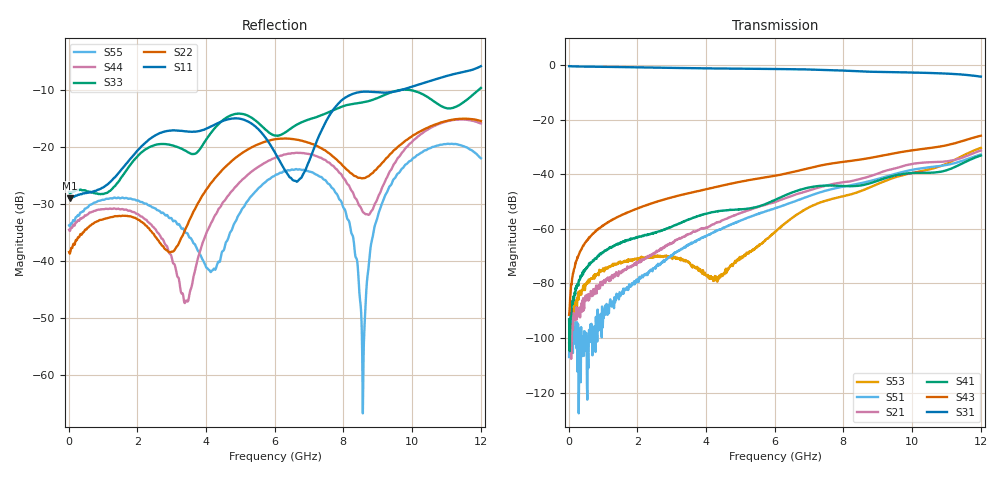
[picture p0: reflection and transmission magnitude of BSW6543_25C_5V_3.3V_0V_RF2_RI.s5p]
! Agilent Technologies	N5230C	MY49001333	A.09.33.09
!	Test time	=	2026-05-28 10:00
!	Product	=	BSW6543
!	Temp	=	25C
!	Logic	=	RF2
!	Port1	=	RFC
!	Port2	=	RF1
!	Port3	=	RF2
!	Port4	=	RF3
!	Port5	=	RF4
!S5P File: Measurements: <S11,S12,S13,S14,S15>,
!<S21,S22,S23,S24,S25>,
!<S31,S32,S33,S34,S35>,
!<S41,S42,S43,S44,S45>,
!<S51,S52,S53,S54,S55>;
# HZ S RI R 50
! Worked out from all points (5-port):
!   1201 points, 10 MHz to 12.01 GHz, reference 50 ohm
!   strongest paths, dB at 10 MHz, 3.01 GHz, 6.01 GHz, 9.01 GHz, 12.01 GHz:
!     S31: -0.5, -1.1, -1.5, -2.6, -4.3
!     S43: -91.5, -48.5, -40.6, -33.5, -25.9
!     S41: -93.2, -59.2, -49.4, -42.4, -33.2
!     S21: -102.0, -65.3, -50.2, -39.8, -31.3
!     S51: -107.0, -69.6, -52.5, -41.8, -32.8
!     S53: -106.6, -70.5, -61.2, -43.5, -30.4
!   lowest |S11| = -29.0 dB at 40 MHz (marker M1), VSWR 1.07, Z = 53.6 - j0.424 ohm
!   |S11| at or under -10 dB: start of sweep to 9.687 GHz
